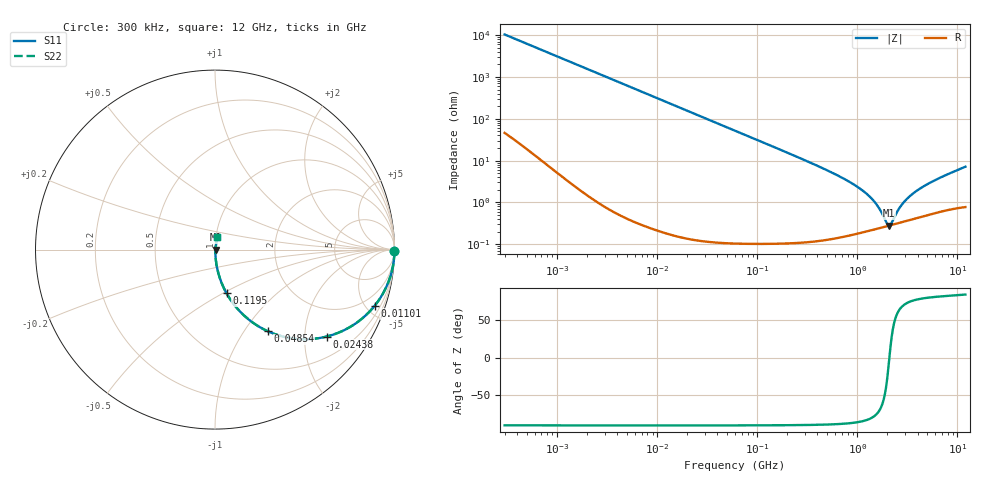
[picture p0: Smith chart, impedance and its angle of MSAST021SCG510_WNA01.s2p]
! MSAST021SCG510_WNA01  S-PARAMETER MODEL  ( Standard Model )
! Model Generated by TAIYO YUDEN Corporation (http://www.ty-top.com)
! Version 2.0
! TAIYO YUDEN Control No. 231201
! Copyright(c) 2023 TAIYO YUDEN CO.,LTD. All Rights Reserved.
! Product Description (link to TY-COMPAS)
! https://ds.yuden.co.jp/TYCOMPAS/or/detail?pn=MSAST021SCG510JWNA01&u=M
! Products Name : Multilayer Ceramic Capacitors
! Characteristics :
!  Capacitance : 51 [pF] , Rated Voltage : 25 [V] , TCC : CG / C0G
!  Case Size : 0.25 x 0.125 / 0.0098 x 0.0049 [mm/inch] , Thickness : 0.125 / 0.0049 [mm/inch]
!  (Conditions: Temperature = 25 [degC] , DC Bias Voltage = 0 [V])
! External Node Assignments :
!  1  o---| |---o  2
! GND o---------o GND
! Frequency Range : 0.3MHz  -  12000MHz  [ 401 STEP ]
# MHZ S RI R 50
! Freq[MHz].  S11 Real  S11 Imag  S21 Real  S21 Imag  S12 Real  S12 Imag  S22 Real  S22 Imag
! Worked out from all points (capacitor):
!   401 points, 300 kHz to 12 GHz, reference 50 ohm
!   read as one part in series: C = 51 pF near 316.3 kHz
!   lowest |Z| = 280 mohm at 2.089 GHz (marker M1)
!   series resonance near 2.089 GHz, so ESL is about 110 pH
!   S11 on the Smith chart (normalised r, x): 300 kHz: open; 11.01 MHz: 1.00, -5.68; 24.38 MHz: 1.00, -2.57; 48.54 MHz: 1.00, -1.29; 119.5 MHz: 1.00, -0.52; 12 GHz: 1.02, +0.14
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0.3  0.9999 -0.00961  0.000135 0.00961  0.000135 0.00961  0.9999 -0.00961
1.769972  0.9967 -0.0564  0.00325 0.0564  0.00325 0.0564  0.9967 -0.0564
4.593584  0.9788 -0.1438  0.0212 0.1438  0.0212 0.1438  0.9788 -0.1438
10.44266  0.8995 -0.3003  0.1005 0.3003  0.1005 0.3003  0.8995 -0.3003
11.01087  0.8896 -0.3131  0.1104 0.3131  0.1104 0.3131  0.8896 -0.3131
16.38321  0.7845 -0.4108  0.2155 0.4108  0.2155 0.4108  0.7845 -0.4108
24.37677  0.622 -0.4844  0.378 0.4844  0.378 0.4844  0.622 -0.4844
34.39878  0.4526 -0.4971  0.5474 0.4971  0.5474 0.4971  0.4526 -0.4971
48.54115  0.2935 -0.4545  0.7065 0.4545  0.7065 0.4545  0.2935 -0.4545
60  0.2139 -0.409  0.7861 0.409  0.7861 0.409  0.2139 -0.409
119.4772  0.0645 -0.2438  0.9355 0.2438  0.9355 0.2438  0.0645 -0.2438
353.9943  0.00837 -0.0847  0.9916 0.0847  0.9916 0.0847  0.00837 -0.0847
743.2595  0.00282 -0.0361  0.9972 0.0361  0.9972 0.0361  0.00282 -0.0361
1166.079  0.00227 -0.0179  0.9977 0.0179  0.9977 0.0179  0.00227 -0.0179
1519.776  0.00237 -0.00932  0.9976 0.00932  0.9976 0.00932  0.00237 -0.00932
1980.756  0.0027 -0.00151  0.9973 0.00151  0.9973 0.00151  0.0027 -0.00151
2088.533  0.00279 1.01e-07  0.9972 -1.01e-07  0.9972 -1.01e-07  0.00279 1.01e-07
2202.174  0.00289 0.0015  0.9971 -0.0015  0.9971 -0.0015  0.00289 0.0015
2795.104  0.00345 0.00826  0.9966 -0.00826  0.9966 -0.00826  0.00345 0.00826
3740.715  0.00438 0.0169  0.9956 -0.0169  0.9956 -0.0169  0.00438 0.0169
6026.253  0.00668 0.0336  0.9933 -0.0336  0.9933 -0.0336  0.00668 0.0336
12000  0.0126 0.0697  0.9874 -0.0697  0.9874 -0.0697  0.0126 0.0697
